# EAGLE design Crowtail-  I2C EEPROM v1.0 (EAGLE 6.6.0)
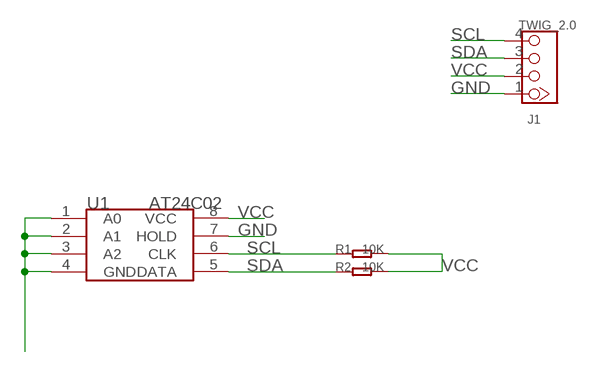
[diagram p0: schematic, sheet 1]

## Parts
J1  TWIG_2.0  [2.0_1X4]
R1  10K  R-0603  [R0603]
R2  10K  R-0603  [R0603]
U1  AT24C02  [SOP8]

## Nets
GND: J1.1 U1.1(A0) U1.2(A1) U1.3(A2) U1.4(GND) U1.7(HOLD)
SCL: J1.4 R1.1 U1.6(CLK)
SDA: J1.3 R2.1 U1.5(DATA)
VCC: J1.2 R1.2 R2.2 U1.8(VCC)

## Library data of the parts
J1 = CONNECTER:TWIG_2.0
R1 R2 = Discrete:R*
U1 = AT24C02:AT24C02

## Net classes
0 default: width 0.203 mm, drill 0.305 mm, clearance 0.203 mm

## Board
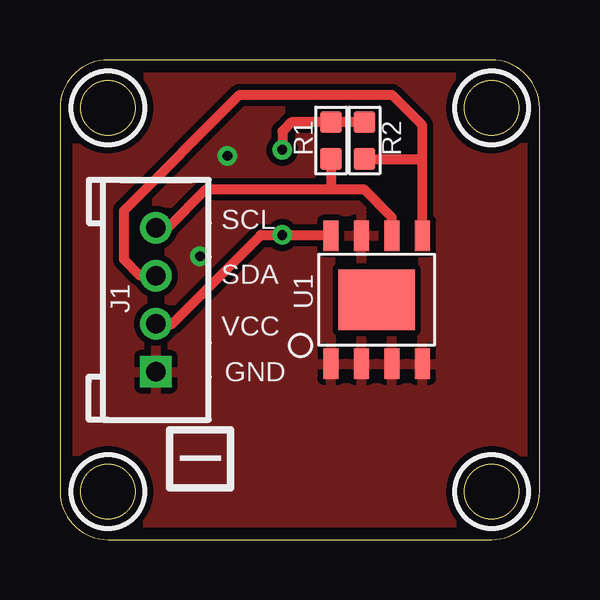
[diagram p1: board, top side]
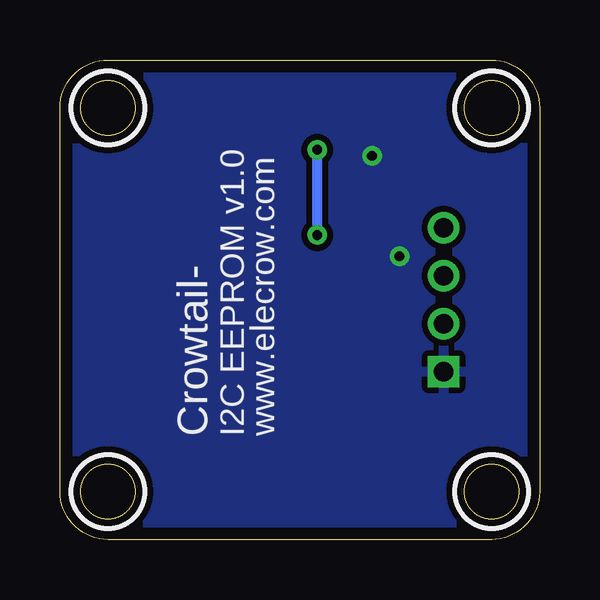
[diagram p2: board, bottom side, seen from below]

Size 20 x 20 mm. Coordinates in mm from the lower left corner, seen from the top.
Outline: 18,20 2,20 arc90 0,18 0,2 arc90 2,0 18,0 arc90 20,2 20,18 arc90 18,20
Outline: circle at 2,18 radius 1.14
Outline: circle at 2,2 radius 1.14
Outline: circle at 18,18 radius 1.14
Outline: circle at 18,2 radius 1.14
Copper layers (1*16): Top 0.035mm / dielectric 1.5mm / Bottom 0.035mm
Design rules: minimum track width 10mil, minimum drill 10mil, track to track 8mil, track to pad 8mil, pad to pad 8mil, via to via 8mil, smd to smd 8mil, copper to edge 20mil, drill to drill 8mil, minimum pad ring 10mil, minimum via ring 8mil, stop-mask expansion 4mil, vias tented up to drill 100mil, thermal gap 10mil
tRestrict: area 0.5,16.5 to 3.5,19.5; area 0.5,0.5 to 3.5,3.5; area 16.5,16.5 to 19.5,19.5; area 16.5,0.5 to 19.5,3.5
bRestrict: area 0.5,16.5 to 3.5,19.5; area 0.5,0.5 to 3.5,3.5; area 16.5,16.5 to 19.5,19.5; area 16.5,0.5 to 19.5,3.5

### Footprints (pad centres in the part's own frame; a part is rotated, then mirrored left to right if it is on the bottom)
2.0_1X4 = drill 0.8 pad 1.27 square: 1 -3,0 | drill 0.8 pad 1.27: 2 -1,0; 3 1,0; 4 3,0
R0603 = smd 0.889 x 0.889: 1 -0.762,0; 2 0.762,0
SOP8 = smd 0.635 x 1.27: 1 -1.905,-2.667; 2 -0.635,-2.667; 3 0.635,-2.667; 4 1.905,-2.667; 5 1.905,2.667; 6 0.635,2.667; 7 -0.635,2.667; 8 -1.905,2.667 | smd 3.175 x 2.54: HEAT 0,0

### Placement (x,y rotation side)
J1  4,10 90 top
R1  11.3,16.64 90 top
R2  12.7,16.64 90 top
U1  13.21,10 0 top

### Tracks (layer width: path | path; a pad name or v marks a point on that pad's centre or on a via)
GND  (via drill 0.41)
  other vias: 6.99,16 5.84,11.81
  pour Bottom (isolate 0.254): 0,0 20.32,0 20.32,20.32 0,20.32
  pour Top (isolate 0.254): 0,0 20.32,0 20.32,20.19 0,20.19
SCL
  Top 0.406: U1.6 13.84,13.43 12.67,14.61 11.3,14.61 | J1.4 4.49,13 6.1,14.61 11.3,14.61 | R1.1 11.3,14.61
SDA
  Top 0.406: J1.3 3.35,11 2.67,11.68 2.67,13.72 7.49,18.54 13.84,18.54 15.11,17.27 15.11,15.88 | U1.5 15.11,15.88 | R2.1 15.11,15.88
VCC  (via drill 0.41)
  Top 0.406: R2.2 R1.2 9.65,17.4 9.27,17.02 v9.27,16.26 | J1.2 4.68,9 8.38,12.7 v9.27,12.7 11.27,12.7 U1.8
  Bottom 0.406: v9.27,16.26 v9.27,12.7

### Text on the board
tPlace: SCL | SDA | VCC | GND | I
bPlace: www.elecrow.com | I2C EEPROM v1.0 | Crowtail-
